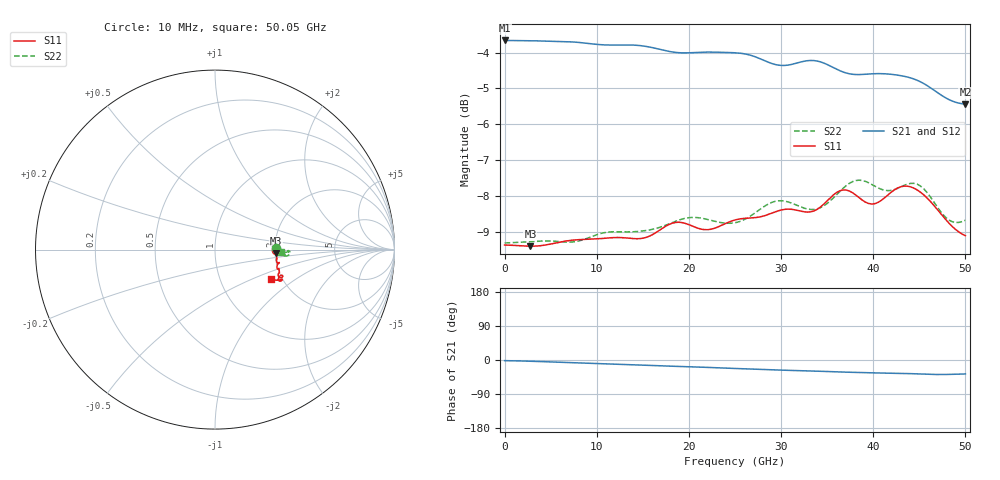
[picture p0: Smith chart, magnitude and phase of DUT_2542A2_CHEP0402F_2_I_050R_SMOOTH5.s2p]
! Touchstone file from project
! Exported from ElectronicsDesktop 2025.1.3
# GHz S MA R 50.000000
! Terminal data exported
! Port[1] = Port1
! Port[2] = Port2
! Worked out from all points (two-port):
!   144 points, 10 MHz to 50.05 GHz, reference 50 ohm
!   highest |S21| = -3.66 dB at 10 MHz (marker M1); lowest = -5.4 dB at 50.05 GHz (marker M2)
!   |S21| within 3 dB of the highest: start of sweep to end of sweep
!   lowest |S11| = -9.4 dB at 2.81 GHz (marker M3), VSWR 2.03, Z = 101 - j4.16 ohm
!   |S11| at or under -10 dB: nowhere
!   |S22| runs from -9.3 to -7.6 dB; largest |S21 - S12| = 0.0076
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0.01  0.3401 -0.2  0.6561 -1.7  0.6565 -1.3  0.3423 1.0
! Gamma 0 0 0 0
! Port Impedance 50 0 50 0
2.8096  0.3388 -3.1  0.6555 -3.2  0.655 -2.9  0.3438 -1.3
4.55935  0.3403 -4.7  0.6547 -4.7  0.6536 -4.5  0.3446 -2.8
8.4088  0.3462 -5.8  0.6513 -7.8  0.6498 -7.7  0.3455 -2.1
11.2084  0.3479 -8.7  0.6466 -10.5  0.6452 -10.3  0.3545 -4.6
14.7079  0.3472 -9.5  0.6454 -13.1  0.6441 -12.9  0.3554 -1.5
16.8076  0.3565 -12.2  0.6379 -15.2  0.637 -15.0  0.3598 -4.1
18.55735  0.3657 -11.8  0.6315 -16.7  0.6311 -16.5  0.367 -4.6
20.3071  0.3618 -11.7  0.6308 -17.9  0.6308 -17.7  0.3716 -3.0
23.45665  0.3617 -16.8  0.6317 -21.0  0.6317 -20.7  0.3656 -4.3
25.2064  0.3691 -17.0  0.6304 -22.6  0.6305 -22.2  0.3657 -5.2
27.3061  0.3715 -16.4  0.622 -24.2  0.6223 -23.9  0.3779 -4.5
29.4058  0.3784 -18.6  0.6073 -26.2  0.6079 -25.8  0.3914 -4.2
33.6052  0.3795 -21.9  0.6151 -29.1  0.6156 -28.8  0.3813 -4.4
35.7049  0.3993 -23.2  0.6015 -31.0  0.6009 -30.8  0.3956 -5.2
38.15455  0.3993 -20.9  0.5881 -32.8  0.5864 -32.5  0.4184 -2.8
39.9043  0.388 -23.9  0.5895 -33.9  0.5879 -33.5  0.4131 -0.9
42.004  0.4031 -25.9  0.5885 -34.8  0.5877 -34.4  0.4054 -1.4
44.45365  0.4083 -24.0  0.5797 -36.3  0.5786 -35.8  0.4146 -2.3
46.2034  0.3918 -25.8  0.5643 -37.9  0.5629 -37.2  0.3977 -2.1
48.3031  0.3645 -27.1  0.5423 -38.0  0.5411 -37.2  0.3683 -2.3
50.05285  0.3504 -27.7  0.5348 -36.9  0.5337 -36.0  0.3683 -2.3
